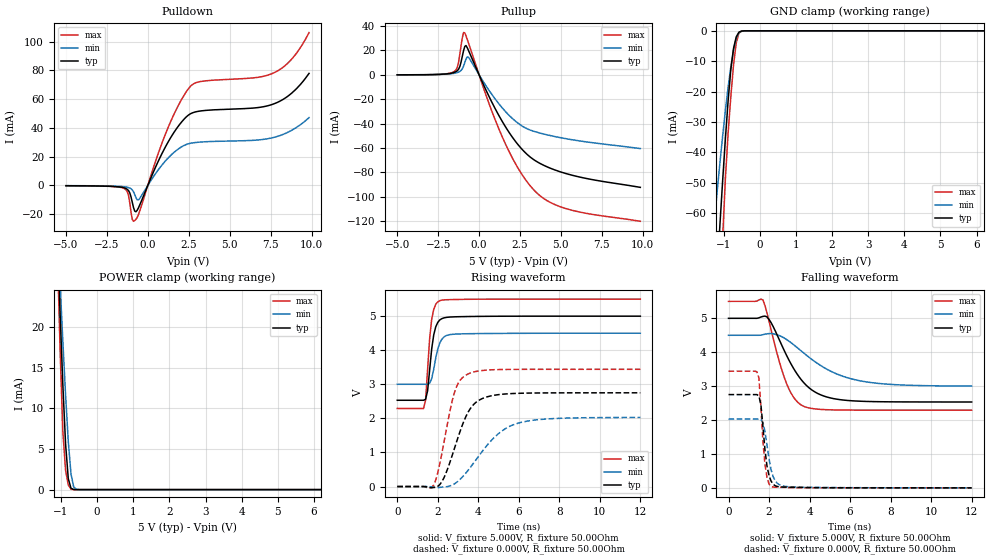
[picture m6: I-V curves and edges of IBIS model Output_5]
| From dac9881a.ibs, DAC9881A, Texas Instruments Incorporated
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[Model]   Output_5
Model_type   3-state
Cref  = 4.5pF   |Timing specification test load capacitance value
Rref  = 5000Ohm
Vref  = 2.5V
Vmeas = 2.5V
|   typ   min   max
|Output tri-stated
C_comp   3.297pF   4.332pF   2.899pF
|Output high
|C_comp   5.174pF   6.279pF   4.294pF
|Output_low
|C_comp   5.429pF   6.137pF   4.771pF
[Voltage Range]   5.000V   4.500V   5.500V
| Junction Temperature (Ambient temp is 25C typ, 105C min,  -40C max)
[Temperature Range]   27.0   105.0   -40.0
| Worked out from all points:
|   slope of the pulldown table from 0 to 0.75 V, typ, clamps not added: 38.4 ohm
|   slope of the pullup table from 0 to 0.75 V, typ, clamps not added: 34.6 ohm
|   GND clamp passes 1 mA (typ) near -0.60 V on its own axis
|   POWER clamp passes 1 mA (typ) near -0.78 V on its own axis
|   falling waveform, V_fixture 5.000V, R_fixture 50.00Ohm: 20-80 % time 1.44ns typ, 2.34ns min, 947ps max; typ from 5 V to 2.53 V
|   rising waveform, V_fixture 5.000V, R_fixture 50.00Ohm: 20-80 % time 290ps typ, 344ps min, 248ps max; typ from 2.53 V to 5 V
|   rising waveform, V_fixture 0.000V, R_fixture 50.00Ohm: 20-80 % time 1.01ns typ, 1.75ns min, 715ps max; typ from 0 V to 2.75 V
|   falling waveform, V_fixture 0.000V, R_fixture 50.00Ohm: 20-80 % time 294ps typ, 357ps min, 245ps max; typ from 2.75 V to 0 V
[Pulldown]
|   Voltage   I(typ)   I(min)   I(max)
-5V       -197.8uA   -148.3uA   -199.3uA
-1.475V   -1.57mA    -882.9uA   -1.991mA
-1.175V   -3.666mA   -1.52mA    -7.133mA
-950mV    -11.72mA   -3.111mA   -23.6mA
-875mV    -15.34mA   -4.404mA   -24.96mA
-725mV    -18.31mA   -8.489mA   -23.55mA
-575mV    -15.65mA   -10.1mA    -20.39mA
1.15V     28.38mA    17.99mA    37.8mA
2.575V    49.68mA    29.25mA    68.62mA
7.675V    56.67mA    33.37mA    78.24mA
8.8V      64.34mA    38.44mA    88.04mA
9.85V     77.99mA    47.19mA    106.4mA
[GND Clamp]
|   Voltage   I(typ)   I(min)   I(max)
-5V       -982.1mA   -692.2mA   -1.337A
-1.325V   -110.1mA   -72.01mA   -157.4mA
-1.25V    -94.15mA   -62.09mA   -134.2mA
-1.1V     -63.57mA   -43.29mA   -89.08mA
-1.025V   -49.12mA   -34.49mA   -67.79mA
-875mV    -23.05mA   -18.58mA   -33.73mA
-800mV    -12.74mA   -11.85mA   -21.67mA
-725mV    -5.794mA   -6.353mA   -11.28mA
-650mV    -1.979mA   -2.491mA   -3.953mA
-575mV    -434.9uA   -630uA     -778.5uA
-500mV    -68.4uA    -133.1uA   -92.74uA
9.85V     0A         0A         0A
[Pullup]
|   Voltage   I(typ)   I(min)   I(max)
-5V       -23.96uA   -11.01uA   -36.93uA
-1.55V    1.794mA    1.145mA    2.434mA
-1.325V   3.42mA     1.818mA    6.319mA
-1.175V   6.796mA    2.74mA     17.09mA
-950mV    19.74mA    7.077mA    34.59mA
-875mV    23.17mA    10.02mA    34.41mA
-650mV    19.99mA    14.43mA    26.11mA
1.375V    -37.28mA   -26.47mA   -49.58mA
2.35V     -56.73mA   -39.35mA   -75.78mA
3.325V    -69.38mA   -46.19mA   -94.02mA
5.275V    -80.76mA   -52.25mA   -109.5mA
9.85V     -92.2mA    -60.44mA   -120mA
[POWER Clamp]
|   Voltage   I(typ)   I(min)   I(max)
-5V       295.4mA    256mA      340.9mA
-1.1V     30.97mA    32.34mA    29.04mA
-1.025V   21.5mA     25.13mA    16.93mA
-950mV    12.84mA    18.17mA    7.113mA
-875mV    5.622mA    11.64mA    2.379mA
-800mV    1.354mA    5.934mA    579.2uA
-725mV    164.8uA    1.934mA    39.25uA
-650mV    12.77uA    323.2uA    2.074uA
-575mV    1.051uA    36.63uA    131.5nA
-500mV    95.89nA    3.929uA    8.344nA
9.85V     0A         0A         0A
[Ramp]
R_load = 50.00Ohm
|   typ   min   max
dV/dt_r   1.650V/1.011ns   1.217V/1.747ns   2.064V/714.683ps
dV/dt_f   1.481V/1.436ns   899.254mV/2.338ns   1.925V/946.803ps
[Falling Waveform]
V_fixture = 5.000V
V_fixture_min = 4.500V
V_fixture_max = 5.500V
R_fixture = 50.00Ohm
|   Time   V(typ)   V(min)   V(max)
0s        5V         4.5V       5.5V
1.7ns     5.057V     4.517V     5.541V
2.1ns     4.873V     4.552V     4.668V
2.5ns     4.376V     4.491V     3.74V
2.8ns     3.988V     4.4V       3.179V
3.2ns     3.534V     4.228V     2.683V
3.7ns     3.112V     3.983V     2.407V
4.7ns     2.709V     3.552V     2.309V
6.5ns     2.555V     3.156V     2.292V
12ns      2.532V     3.001V     2.291V
[Rising Waveform]
V_fixture = 5.000V
V_fixture_min = 4.500V
V_fixture_max = 5.500V
R_fixture = 50.00Ohm
|   Time   V(typ)   V(min)   V(max)
0s        2.532V     3.001V     2.291V
1.3ns     2.532V     3.001V     2.291V
1.4ns     2.561V     3.001V     2.539V
1.5ns     2.815V     3V         3.45V
1.6ns     3.425V     3.032V     4.351V
1.7ns     4.037V     3.168V     4.906V
1.9ns     4.686V     3.771V     5.349V
2.1ns     4.889V     4.212V     5.456V
2.9ns     4.982V     4.474V     5.489V
12ns      5V         4.5V       5.5V
[Rising Waveform]
V_fixture = 0.000V
V_fixture_min = 0.000V
V_fixture_max = 0.000V
R_fixture = 50.00Ohm
|   Time   V(typ)   V(min)   V(max)
0s        -6.282uV   13.08uV    -18.17uV
1.8ns     -28.52mV   -19.4mV    44.98mV
2.2ns     139.2mV    -17.94mV   966mV
2.8ns     1.074V     69.8mV     2.714V
3.1ns     1.617V     209.7mV    3.117V
3.5ns     2.185V     478.3mV    3.305V
4.3ns     2.606V     1.112V     3.412V
5.1ns     2.704V     1.601V     3.434V
5.9ns     2.734V     1.847V     3.439V
12ns      2.751V     2.028V     3.44V
[Falling Waveform]
V_fixture = 0.000V
V_fixture_min = 0.000V
V_fixture_max = 0.000V
R_fixture = 50.00Ohm
|   Time   V(typ)   V(min)   V(max)
0s        2.751V     2.028V     3.44V
1.4ns     2.751V     2.028V     3.425V
1.5ns     2.711V     2.029V     3.24V
1.6ns     2.446V     2.016V     2.38V
1.7ns     1.802V     1.927V     1.355V
1.8ns     1.115V     1.659V     694.2mV
2.1ns     200.2mV    539.6mV    40.79mV
2.4ns     41.33mV    139.1mV    19.31mV
2.9ns     20.52mV    36.97mV    10.95mV
12ns      -6.282uV   13.08uV    -18.17uV
